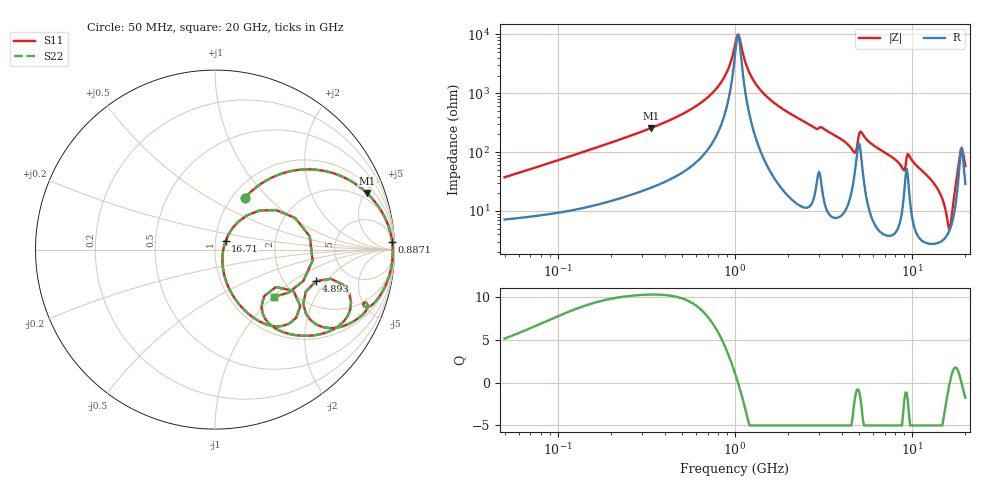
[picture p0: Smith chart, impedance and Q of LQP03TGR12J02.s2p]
!Murata Part Number: LQP03TGR12J02
!These Parameters are Measured in Series Mode Connection
!  o--[Z]--o
!Port1  Port2
!  o-------o
!Freq. Start=50[MHz] Stop=20[GHz], 401[Steps]
# Hz S RI R 50
!Freq.(Hz) S11(Real) S11(Imag) S21(Real) S21(Imag) S12(Real) S12(Imag) S22(Real) S22(Imag)
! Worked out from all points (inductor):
!   401 points, 50 MHz to 20 GHz, reference 50 ohm
!   read as one part in series: L = 116 nH near 51.52 MHz
!   highest Q = 10.3 at 335.1 MHz (marker M1), where L = 121 nH
!   self-resonance near 1.03 GHz
!   S11 on the Smith chart (normalised r, x): 50 MHz: 1.14, +0.74; 887.1 MHz: 11, +41; 4.893 GHz: 2.94, -1.59; 16.71 GHz: 1.12, +0.10; 20 GHz: 1.58, -1.01
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5e7  0.1654 0.2867  0.8346 -0.2867  0.8346 -0.2867  0.1654 0.2867
1.364002e8  0.4958 0.4466  0.5042 -0.4466  0.5042 -0.4466  0.4958 0.4466
3.350611e8  0.8456 0.3159  0.1544 -0.3159  0.1544 -0.3159  0.8456 0.3159
3.721004e8  0.8726 0.2883  0.1274 -0.2883  0.1274 -0.2883  0.8726 0.2883
6.574395e8  0.9665 0.1296  0.0335 -0.1296  0.0335 -0.1296  0.9665 0.1296
8.870719e8  0.9865 0.045  0.0135 -0.045  0.0135 -0.045  0.9865 0.045
1e9  0.9897 0.011  0.0103 -0.011  0.0103 -0.011  0.9897 0.011
1.061746e9  0.9904 -0.00614  0.00964 0.00614  0.00964 0.00614  0.9904 -0.00614
1.196911e9  0.9896 -0.0408  0.0104 0.0408  0.0104 0.0408  0.9896 -0.0408
1.454215e9  0.9822 -0.0986  0.0178 0.0986  0.0178 0.0986  0.9822 -0.0986
2.728004e9  0.8724 -0.3096  0.1276 0.3096  0.1276 0.3096  0.8724 -0.3096
4.34015e9  0.6344 -0.4368  0.3656 0.4368  0.3656 0.4368  0.6344 -0.4368
4.89267e9  0.5636 -0.1756  0.4364 0.1756  0.4364 0.1756  0.5636 -0.1756
5.273168e9  0.7541 -0.3308  0.2459 0.3308  0.2459 0.3308  0.7541 -0.3308
7.442007e9  0.4404 -0.4754  0.5596 0.4754  0.5596 0.4754  0.4404 -0.4754
9.178299e9  0.3386 -0.2087  0.6614 0.2087  0.6614 0.2087  0.3386 -0.2087
1.220001e10  0.1526 -0.3256  0.8474 0.3256  0.8474 0.3256  0.1526 -0.3256
1.438523e10  0.063 -0.179  0.937 0.179  0.937 0.179  0.063 -0.179
1.597544e10  0.0418 -0.039  0.9582 0.039  0.9582 0.039  0.0418 -0.039
1.670968e10  0.0585 0.0462  0.9415 -0.0462  0.9415 -0.0462  0.0585 0.0462
1.855685e10  0.4463 0.1764  0.5537 -0.1764  0.5537 -0.1764  0.4463 0.1764
2e10  0.3266 -0.2631  0.6734 0.2631  0.6734 0.2631  0.3266 -0.2631
